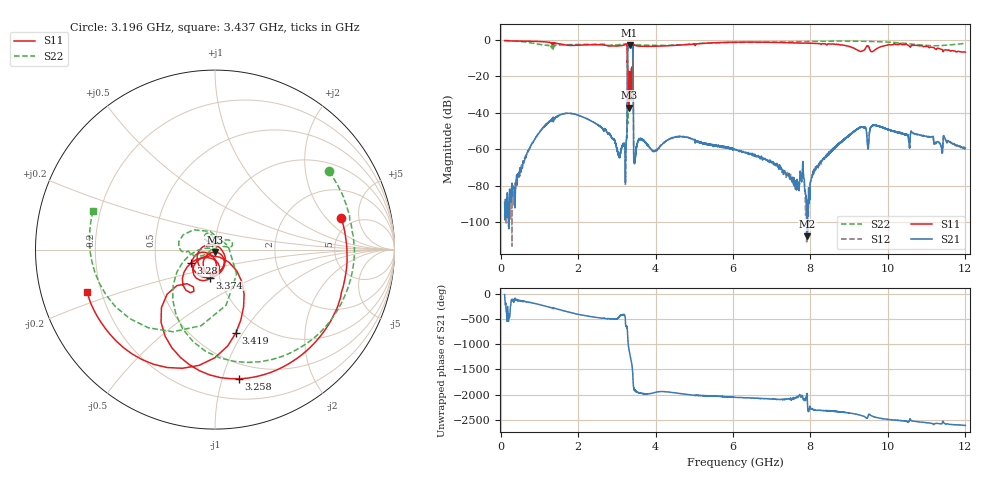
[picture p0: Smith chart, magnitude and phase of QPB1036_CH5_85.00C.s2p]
! TDS: K:\Engsetup\Winsaw\QPB1036_ALL
! Channel 1
! Ports=1 2
! seg 1=100.000000 1100.000000 101
! seg 2=1101.000000 1501.000000 401
! seg 3=1502.000000 2502.000000 101
! seg 4=2503.000000 3803.000000 1301
! seg 5=3804.000000 5004.000000 121
! seg 6=5005.000000 6005.000000 1001
! seg 7=6006.000000 8406.000000 241
! seg 8=8407.000000 10607.000000 2201
! seg 9=10608.000000 12008.000000 141
! Points=5609
! FailCode=0
! Topology=ALL_SE(12)
!VNA Cal loaded =QPB1036_ALL_85C
!PS1(V)= 5.000
!PS(mA)= 0.600
!PS2(V)= 1.170
!PS(mA)= -0.100
!PS3(V)= 0.630
!PS(mA)= 0.100
!PS4(V)= 1.170
!PS(mA)= -0.100
!Temp (C)= 85.00
# MHz S DB R 50
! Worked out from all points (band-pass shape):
!   5609 points, 100 MHz to 12.01 GHz, reference 50 ohm
!   highest |S21| = -2.78 dB at 3.331 GHz (marker M1); lowest = -107.8 dB at 7.926 GHz (marker M2)
!   |S21| within 3 dB of the highest: 3.283 GHz to 3.413 GHz (129.6 MHz wide, 3.87 % of centre)
!   lowest |S11| = -37.1 dB at 3.312 GHz (marker M3), VSWR 1.03, Z = 49.8 - j1.38 ohm
!   |S11| at or under -10 dB: 3.27 GHz to 3.416 GHz (146.7 MHz wide, 4.39 % of centre)
!   |S22| runs from -46.0 to -0.3 dB; largest |S21 - S12| = 0.0085
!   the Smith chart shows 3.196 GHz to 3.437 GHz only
!   S11 on the Smith chart (normalised r, x): 3.196 GHz: 3.94, +2.96; 3.258 GHz: 0.37, -1.13; 3.28 GHz: 0.76, -0.12; 3.374 GHz: 0.90, -0.29; 3.419 GHz: 0.78, -0.93; 3.437 GHz: 0.15, -0.16
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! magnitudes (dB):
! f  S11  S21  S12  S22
! 100 MHz  -0.4  -89.1  -95.8  -0.3
! 1.233 GHz  -1.3  -45.3  -45.2  -3.0
! 2.092 GHz  -2.8  -42.0  -42.1  -2.5
! 3.196 GHz  -2.8  -57.2  -57.4  -2.3
! 3.237 GHz  -2.4  -58.9  -59.3  -2.2
! 3.258 GHz  -2.7  -53.2  -53.0  -2.6
! 3.28 GHz  -16.3  -7.0  -7.0  -29.2
! 3.312 GHz  -37.1  -3.1  -3.1  -23.2
! 3.331 GHz  -17.5  -2.8  -2.8  -29.1
! 3.374 GHz  -16.0  -3.1  -3.0  -22.7
! 3.398 GHz  -19.7  -3.6  -3.6  -27.4
! 3.419 GHz  -6.4  -10.7  -10.7  -22.3
! 3.437 GHz  -2.5  -67.2  -64.9  -2.9
! 3.463 GHz  -2.8  -66.7  -66.3  -2.8
! 3.589 GHz  -3.5  -54.2  -54.4  -2.8
! 4.074 GHz  -3.4  -59.5  -59.5  -3.0
! 6.056 GHz  -1.3  -60.1  -60.4  -1.4
! 7.926 GHz  -1.8  -107.8  -90.9  -0.9
! 8.046 GHz  -1.9  -75.4  -73.8  -0.8
! 9.267 GHz  -6.0  -48.2  -48.2  -0.7
! 10.02 GHz  -2.6  -49.2  -49.2  -1.3
! 12.01 GHz  -6.7  -59.4  -59.0  -2.0
